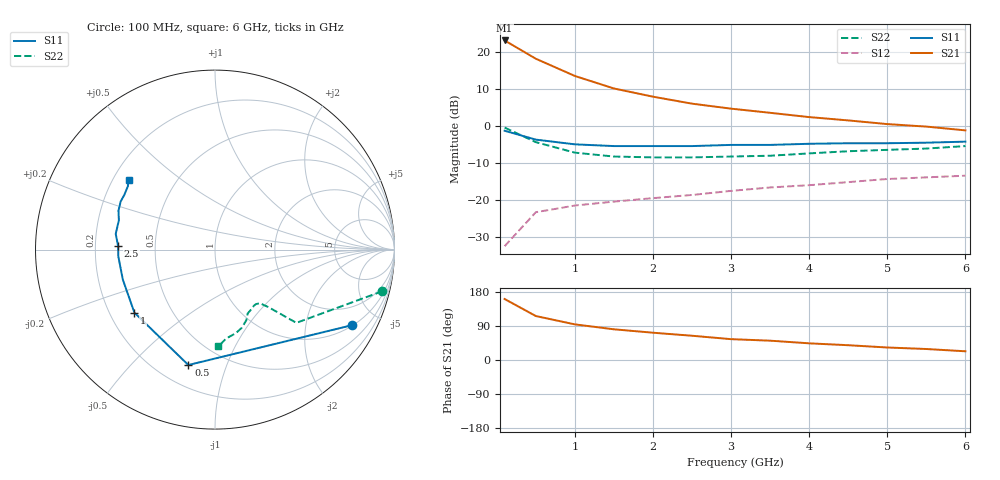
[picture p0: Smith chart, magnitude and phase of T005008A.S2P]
!AT-00500
!S-PARAMETERS at Vce=8 V  Ic=5 mA.
!OBSOLETED Feb 1994 - nearest replacement: AT-41400
# ghz s ma r 50
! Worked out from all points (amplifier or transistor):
!   13 points, 100 MHz to 6 GHz, reference 50 ohm
!   highest |S21| = 23.2 dB at 100 MHz (marker M1)
!   |S21| within 3 dB of that: start of sweep to 342.9 MHz
!   unconditionally stable (mu >= 1): 1.782 GHz to 5.744 GHz
!   at 1 GHz: K = 0.67, MSG = 17.5 dB, |S12| = -21.4 dB
!   at 3 GHz: K = 1.15, MAG = 8.7 dB, |S12| = -17.5 dB
!   at 6 GHz: K = 0.97, MSG = 6.1 dB, |S12| = -13.4 dB
!   S11 on the Smith chart (normalised r, x): 100 MHz: 1.03, -3.59; 500 MHz: 0.33, -0.74; 1 GHz: 0.30, -0.32; 2.5 GHz: 0.30, +0.02; 6 GHz: 0.26, +0.33
0.1  0.87 -29.0  14.43 161.0  0.024 76.0  0.96 -14.0
0.5  0.66 -103.0  8.17 116.0  0.069 45.0  0.61 -42.0
1  0.57 -142.0  4.78 94.0  0.085 40.0  0.44 -47.0
1.5  0.54 -162.0  3.24 81.0  0.096 44.0  0.39 -50.0
2  0.54 -176.0  2.51 72.0  0.107 49.0  0.38 -53.0
2.5  0.54 178.0  2.02 64.0  0.118 52.0  0.38 -55.0
3  0.56 171.0  1.73 55.0  0.134 53.0  0.39 -59.0
3.5  0.56 163.0  1.52 51.0  0.149 58.0  0.4 -63.0
4  0.58 158.0  1.33 44.0  0.16 59.0  0.43 -66.0
4.5  0.59 153.0  1.2 39.0  0.176 60.0  0.46 -71.0
5  0.59 149.0  1.07 33.0  0.194 61.0  0.48 -76.0
5.5  0.6 144.0  0.99 29.0  0.204 62.0  0.5 -83.0
6  0.62 141.0  0.88 23.0  0.215 63.0  0.54 -88.0
